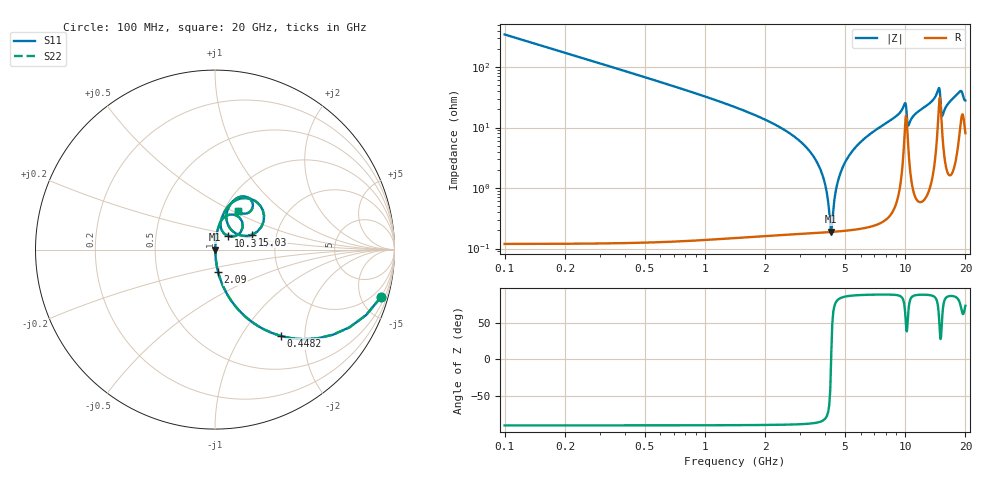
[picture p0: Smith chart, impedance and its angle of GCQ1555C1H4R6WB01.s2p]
!Murata Part Number: GCQ1555C1H4R6WB01
!These Parameters are Measured in Series Mode Connection
!Data Generated on Mar 13, 2026
!  o--ll--o
!Port1  Port2
!  o------o
!Operation Temp=25[degC], DC Bias Voltage=0[V]
!Freq. Start=100[MHz] Stop=20[GHz] 401[Steps]
# Hz S RI R 50
!Freq.(Hz) S11(Real) S11(Imag) S21(Real) S21(Imag) S12(Real) S12(Imag) S22(Real) S22(Imag)
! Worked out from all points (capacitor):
!   401 points, 100 MHz to 20 GHz, reference 50 ohm
!   read as one part in series: C = 4.6 pF near 199.5 MHz
!   lowest |Z| = 190 mohm at 4.279 GHz (marker M1)
!   series resonance near 4.272 GHz, so ESL is about 300 pH
!   S11 on the Smith chart (normalised r, x): 100 MHz: 1.00, -6.92; 448.2 MHz: 1.00, -1.53; 2.09 GHz: 1.00, -0.25; 10.3 GHz: 1.14, +0.18; 15.03 GHz: 1.49, +0.26; 20 GHz: 1.16, +0.54
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1e8  0.9227 -0.2668  0.0773 0.2668  0.0773 0.2668  0.9227 -0.2668
4.4825e8  0.3684 -0.4815  0.6316 0.4815  0.6316 0.4815  0.3684 -0.4815
9.4575e8  0.1089 -0.3096  0.8911 0.3096  0.8911 0.3096  0.1089 -0.3096
2.09e9  0.0172 -0.1237  0.9828 0.1237  0.9828 0.1237  0.0172 -0.1237
3.43325e9  0.00307 -0.0358  0.9969 0.0358  0.9969 0.0358  0.00307 -0.0358
3.93075e9  0.00203 -0.0136  0.998 0.0136  0.998 0.0136  0.00203 -0.0136
4.1795e9  0.00188 -0.00357  0.9981 0.00357  0.9981 0.00357  0.00188 -0.00357
4.279e9  0.00188 0.000271  0.9981 -0.000271  0.9981 -0.000271  0.00188 0.000271
4.5775e9  0.00204 0.0113  0.998 -0.0113  0.998 -0.0113  0.00204 0.0113
4.9755e9  0.00259 0.0251  0.9974 -0.0251  0.9974 -0.0251  0.00259 0.0251
5.672e9  0.00432 0.0474  0.9957 -0.0474  0.9957 -0.0474  0.00432 0.0474
6.7665e9  0.00871 0.0797  0.9913 -0.0797  0.9913 -0.0797  0.00871 0.0797
9.40325e9  0.0387 0.1667  0.9613 -0.1667  0.9613 -0.1667  0.0387 0.1667
1.005e10  0.1514 0.156  0.8486 -0.156  0.8486 -0.156  0.1514 0.156
1.029875e10  0.0717 0.0764  0.9283 -0.0764  0.9283 -0.0764  0.0717 0.0764
1.338325e10  0.0718 0.2381  0.9282 -0.2381  0.9282 -0.2381  0.0718 0.2381
1.467675e10  0.2362 0.2618  0.7638 -0.2618  0.7638 -0.2618  0.2362 0.2618
1.5025e10  0.2069 0.0832  0.7931 -0.0832  0.7931 -0.0832  0.2069 0.0832
1.53235e10  0.0899 0.1114  0.9101 -0.1114  0.9101 -0.1114  0.0899 0.1114
1.67165e10  0.0796 0.2421  0.9204 -0.2421  0.9204 -0.2421  0.0796 0.2421
1.8806e10  0.1881 0.2876  0.8119 -0.2876  0.8119 -0.2876  0.1881 0.2876
2e10  0.1285 0.2166  0.8715 -0.2166  0.8715 -0.2166  0.1285 0.2166
